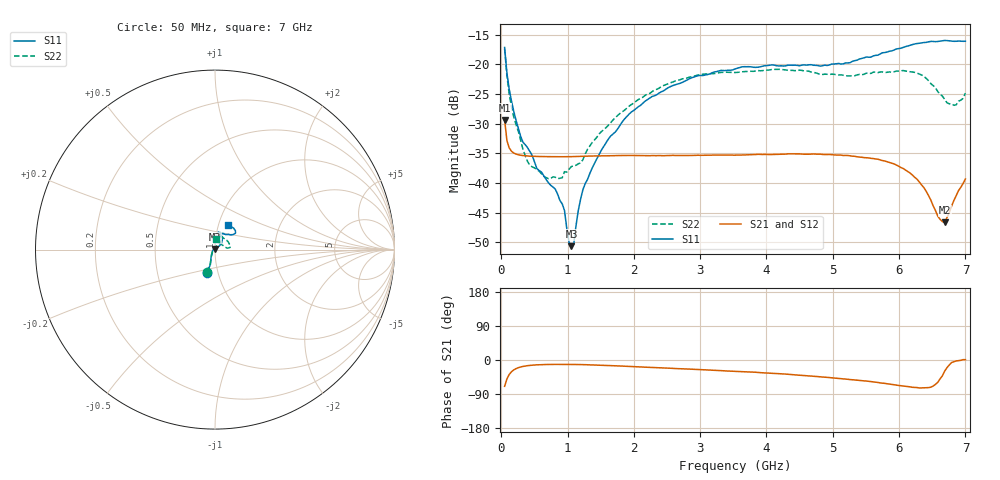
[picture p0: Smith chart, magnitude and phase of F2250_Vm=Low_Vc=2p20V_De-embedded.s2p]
! Integrated Device Technology
! Corporate Headquarters
! 6024 Silver Creek Valley Road
! San Jose, CA 95138  USA
! Phone:  1-408-284-8200
! Toll Free:  1-800-223-1366
! Webpage:  http://www.idt.com/
! Timing and RF Division
! 515 Groton Road, Suite 102
! Westford, MA 01886-6024
! Device:  F2250
! Description: Voltage Variable RF Attenuator
! Frequency:  50.0 -  6000.00 MHz
! Package:  3x3 mm Thin QFN Plastic Package: 16 pin
! Ports:  2 RF, 3 DC
!  Pin  1  = GND
!  Pin  2  = NC
!  Pin  3  = RF1  = Port 1
!  Pin  4  = NC
!  Pin  5  = GND
!  Pin  6  = GND
!  Pin  7  = GND
!  Pin  8  = GND
!  Pin  9  = NC
!  Pin 10  = RF2  = Port 2
!  Pin 11  = NC
!  Pin 12  = GND
!  Pin 13  = GND
!  Pin 14  = VCNTRL
!  Pin 15  = VDD
!  Pin 16  = VMODE
! Vcntrl:  2.200 Volts
! Vmode:  +0.000 Volts
! Vdd:  +3.30  Volts
! Current:  1.179 mA
! Data:  The device was measured on a the F2250 evaluation board which has
!  individual transmission lines to the RF pins.  Data was collected
!  using a calibrated network analyzer.  The evaluation board was
!  de-embedded using a TRL calibration technique.
!  The reference plane is the edge of the package pin.
! Misc:  SN 10
!  Action Tracker AT0258
! Date Measured:  2014-11-26
! Date:  2015-10-15  MJV
! Note:
!  Integrated Device Technology supplies this data as a sample of measured
!  data at the package pin for this product.  Your particular data for this
!  product may vary.
!  Data was taken at 25 degrees C.
!  Integrated Device Technology reserves the right to change this data at anytime.
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# GHz S dB R 50
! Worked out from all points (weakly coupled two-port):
!   201 points, 50 MHz to 7 GHz, reference 50 ohm
!   highest |S21| = -29.38 dB at 50 MHz (marker M1); lowest = -46.7 dB at 6.687 GHz (marker M2)
!   lowest |S11| = -50.7 dB at 1.058 GHz (marker M3), VSWR 1.01, Z = 49.8 + j0.244 ohm
!   |S11| at or under -10 dB: start of sweep to end of sweep
!   |S22| runs from -39.3 to -17.4 dB; largest |S21 - S12| = 6.2e-05
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0.05  -17.18 -108.6  -29.38 -69.4  -29.38 -69.4  -17.40 -110.4
0.08475  -21.44 -107.4  -32.85 -50.0  -32.85 -50.0  -21.94 -108.7
0.15425  -26.23 -116.6  -34.67 -30.9  -34.67 -30.9  -27.17 -119.6
0.29325  -32.20 -127.7  -35.34 -18.3  -35.34 -18.4  -32.85 -132.8
0.3975  -34.08 -141.7  -35.46 -14.9  -35.46 -14.9  -36.41 -156.5
0.6755  -39.41 -163.8  -35.57 -11.9  -35.57 -11.9  -39.10 156.9
0.91875  -43.53 158.1  -35.59 -11.6  -35.58 -11.6  -39.14 125.8
0.9535  -44.67 169.9  -35.59 -11.6  -35.58 -11.6  -38.11 124.0
1.023  -50.04 144.0  -35.58 -11.6  -35.58 -11.6  -37.68 106.8
1.05775  -50.66 123.2  -35.57 -11.7  -35.57 -11.7  -37.23 101.4
1.0925  -50.31 90.3  -35.56 -11.8  -35.56 -11.8  -37.13 96.5
1.162  -44.61 56.9  -35.54 -11.9  -35.54 -12.0  -36.78 85.3
1.2315  -41.11 44.2  -35.52 -12.2  -35.51 -12.2  -36.07 76.1
1.6485  -32.12 41.9  -35.42 -14.7  -35.43 -14.7  -29.88 59.6
2.37825  -24.87 47.3  -35.39 -20.4  -35.39 -20.5  -24.04 54.4
3.525  -20.80 72.5  -35.32 -29.8  -35.32 -29.8  -21.39 73.6
4.7065  -20.17 72.4  -35.12 -42.8  -35.13 -42.8  -21.40 71.6
5.85325  -17.82 40.5  -36.56 -63.5  -36.55 -63.5  -21.29 21.7
6.27025  -16.50 40.1  -39.37 -72.7  -39.38 -72.8  -21.49 8.4
6.68725  -15.99 48.8  -46.67 -29.4  -46.65 -29.2  -25.94 27.4
6.861  -16.13 55.1  -42.16 -2.6  -42.12 -2.7  -26.83 58.0
7  -16.12 63.3  -39.34 0.8  -39.30 0.7  -24.88 83.9
